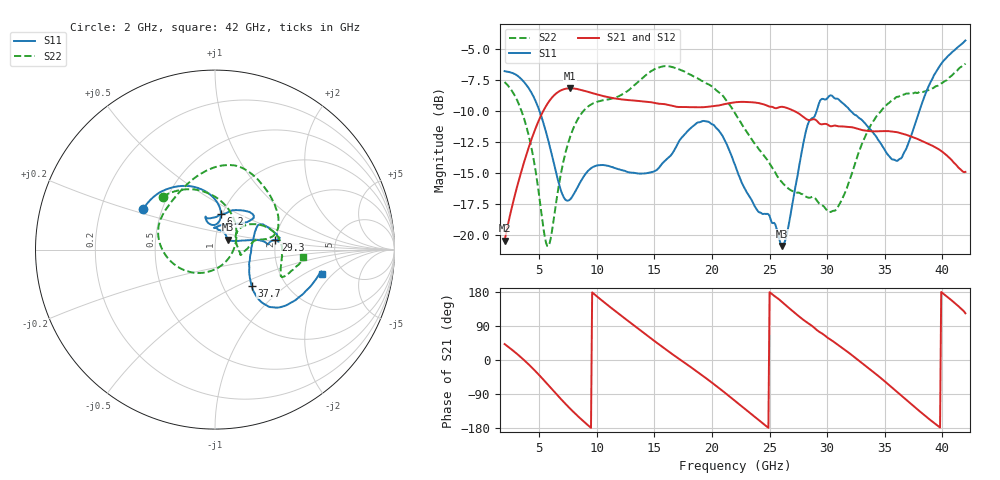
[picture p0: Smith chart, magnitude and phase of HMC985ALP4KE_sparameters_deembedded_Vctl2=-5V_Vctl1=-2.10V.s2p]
!s2p File: Measurements: S11, S21, S12, S22
# GHz S dB R 50.0
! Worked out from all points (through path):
!   401 points, 2 GHz to 42 GHz, reference 50 ohm
!   highest |S21| = -8.15 dB at 7.7 GHz (marker M1); lowest = -20.5 dB at 2 GHz (marker M2)
!   lowest |S11| = -20.9 dB at 26.1 GHz (marker M3), VSWR 1.20, Z = 57.2 + j6.48 ohm
!   |S11| at or under -10 dB: 5.035 GHz to 29.08 GHz (24.04 GHz wide, 141 % of centre); 32.06 GHz to 38 GHz (5.937 GHz wide, 16.9 % of centre)
!   |S22| runs from -20.9 to -6.1 dB; largest |S21 - S12| = 0.00043
!   S11 on the Smith chart (normalised r, x): 2 GHz: 0.39, +0.23; 6.2 GHz: 0.98, +0.41; 29.3 GHz: 2.00, +0.24; 37.7 GHz: 1.36, -0.60; 42 GHz: 3.47, -1.48
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2  -6.76 150.3  -20.48 42.0  -20.48 42.0  -7.63 134.6
3.3  -7.26 129.6  -15.38 10.3  -15.38 10.3  -9.58 101.8
4.6  -8.99 105.2  -11.60 -27.0  -11.60 -27.0  -14.32 55.6
5.6  -11.71 86.8  -9.57 -59.6  -9.58 -59.6  -20.67 -21.8
6.2  -13.92 80.6  -8.80 -80.0  -8.81 -80.0  -19.18 -90.0
7.7  -17.13 97.4  -8.14 -128.7  -8.15 -128.7  -12.05 -163.3
8.7  -15.54 106.4  -8.29 -157.7  -8.29 -157.7  -10.15 173.0
10.2  -14.37 106.0  -8.69 163.2  -8.69 163.2  -9.19 150.8
12.2  -14.78 104.8  -9.04 115.2  -9.05 115.2  -8.64 125.8
15.4  -14.58 85.8  -9.39 41.3  -9.39 41.3  -6.46 81.9
18.5  -11.10 49.7  -9.69 -26.2  -9.69 -26.1  -7.22 47.6
22  -14.35 48.9  -9.28 -108.1  -9.28 -108.0  -10.15 12.0
24.1  -18.19 89.5  -9.35 -159.5  -9.35 -159.4  -13.12 12.2
26.1  -20.91 38.6  -9.64 152.7  -9.65 152.7  -15.78 -3.8
28.7  -10.56 5.4  -10.67 89.7  -10.67 89.7  -16.93 -7.8
29.3  -9.34 9.1  -10.98 74.7  -10.98 74.7  -17.47 -3.1
30.8  -8.98 13.0  -11.19 42.8  -11.19 42.8  -17.97 25.2
32.4  -10.29 26.3  -11.36 6.8  -11.36 6.8  -14.32 40.2
35.4  -13.65 6.9  -11.62 -66.7  -11.62 -66.7  -9.31 16.4
37.7  -10.87 -44.6  -12.19 -126.8  -12.20 -126.7  -8.50 -6.4
39.8  -6.30 -41.5  -13.16 -178.3  -13.16 -178.2  -7.79 -22.0
42  -4.27 -12.6  -14.91 123.2  -14.91 123.2  -6.14 -4.5
